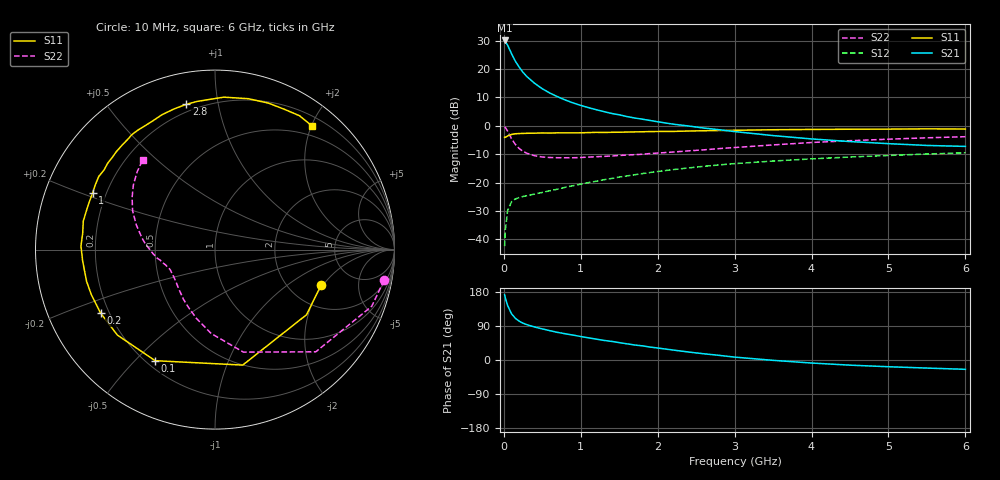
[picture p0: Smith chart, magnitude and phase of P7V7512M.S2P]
! SIEMENS Small Signal Semiconductors
! BFP196
! Si NPN RF Bipolar Junction Transistor in SOT143
! VCE = 0.75 V  IC = 12 mA
! Common Emitter S-Parameters:  May  1996
# GHz  S  MA  R  50
!  f  S11  S21  S12  S22
! GHz  MAG  ANG  MAG  ANG  MAG  ANG  MAG  ANG
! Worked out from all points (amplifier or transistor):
!   36 points, 10 MHz to 6 GHz, reference 50 ohm
!   highest |S21| = 30.0 dB at 10 MHz (marker M1)
!   |S21| within 3 dB of that: start of sweep to 71.93 MHz
!   unconditionally stable (mu >= 1): 779.5 MHz to end of sweep
!   at 250 MHz: K = 0.47, MSG = 21.8 dB, |S12| = -24.9 dB
!   at 1.4 GHz: K = 1.16, MAG = 9.0 dB, |S12| = -18.6 dB
!   at 6 GHz: K = 1.03, MAG = 0.0 dB, |S12| = -9.5 dB
!   S11 on the Smith chart (normalised r, x): 10 MHz: 2.96, -1.92; 100 MHz: 0.23, -0.57; 200 MHz: 0.17, -0.25; 1 GHz: 0.15, +0.22; 2.8 GHz: 0.16, +0.81; 6 GHz: 0.34, +2.00
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0.01  0.6232 -18.5  31.69 172.4  0.0076 84.4  0.9577 -10.3
0.02  0.626 -35.4  30.36 163.4  0.015 74.4  0.9285 -19.9
0.05  0.6617 -76.5  26.04 143.3  0.0324 57.4  0.7997 -45.4
0.1  0.703 -118.3  18.54 121.9  0.046 41.2  0.5927 -74.5
0.15  0.7229 -138.8  13.64 110.0  0.0515 34.3  0.4681 -92.6
0.2  0.7289 -151.0  10.72 102.4  0.0546 31.4  0.3971 -105.1
0.25  0.7334 -160.0  8.684 97.1  0.0571 30.7  0.3525 -115.1
0.3  0.737 -166.1  7.331 93.2  0.0587 30.8  0.3276 -122.5
0.4  0.74 -175.0  5.582 87.1  0.0629 32.2  0.2968 -133.1
0.5  0.7471 178.5  4.481 82.1  0.0671 34.4  0.282 -140.5
0.6  0.7428 172.9  3.752 77.3  0.0719 36.7  0.2758 -145.8
0.7  0.7508 167.8  3.235 72.8  0.0766 38.1  0.2737 -149.8
0.8  0.7486 163.8  2.835 69.2  0.0826 39.4  0.2735 -152.9
1  0.7511 155.2  2.281 62.0  0.0937 41.5  0.276 -157.4
1.1  0.7581 151.7  2.083 58.4  0.0998 42.2  0.2808 -159.3
1.6  0.7747 135.1  1.45 42.7  0.1309 42.2  0.3054 -167.2
2.2  0.7946 117.0  1.067 26.3  0.1691 38.1  0.3446 -175.9
2.8  0.8253 101.2  0.851 12.2  0.2045 32.0  0.3964 173.9
3.5  0.8507 86.7  0.671 -0.9  0.2393 23.7  0.46 162.5
4.5  0.8686 70.0  0.527 -13.6  0.2817 12.6  0.5458 147.8
5.5  0.8821 57.7  0.45 -21.3  0.318 1.9  0.6133 135.0
6  0.8756 52.1  0.433 -24.6  0.3345 -4.0  0.6418 128.9
